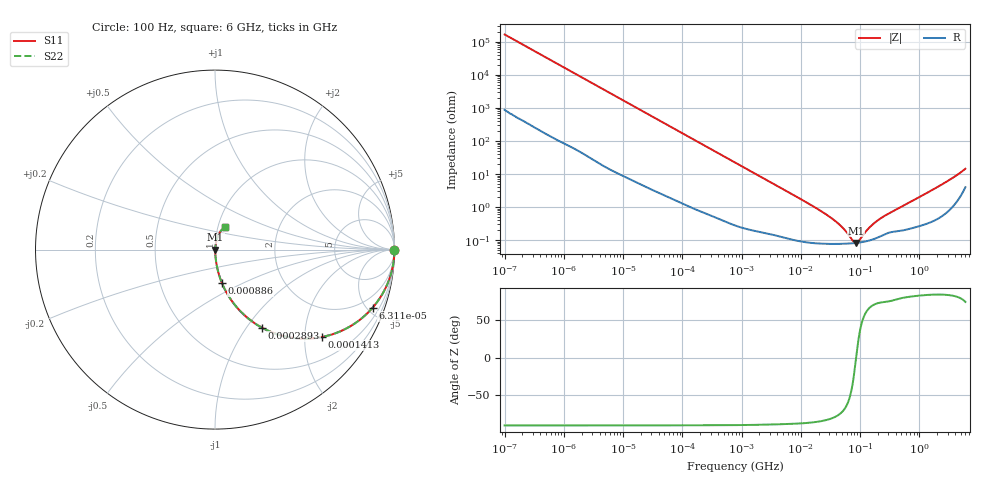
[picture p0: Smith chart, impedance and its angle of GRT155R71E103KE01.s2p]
!Murata Part Number: GRT155R71E103KE01
!These Parameters are Measured in Series Mode Connection
!Data Generated on Jun 19, 2026
!  o--ll--o
!Port1  Port2
!  o------o
!Operation Temp=25[degC], DC Bias Voltage=0[V]
!Freq. Start=100[Hz] Stop=6[GHz] 401[Steps]
# Hz S RI R 50
!Freq.(Hz) S11(Real) S11(Imag) S21(Real) S21(Imag) S12(Real) S12(Imag) S22(Real) S22(Imag)
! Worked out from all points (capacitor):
!   401 points, 100 Hz to 6 GHz, reference 50 ohm
!   read as one part in series: C = 9.51 nF near 109 Hz
!   lowest |Z| = 82.6 mohm at 85.28 MHz (marker M1)
!   series resonance near 85.79 MHz, so ESL is about 360 pH
!   S11 on the Smith chart (normalised r, x): 100 Hz: open; 63.12 kHz: 1.04, -5.41; 141.3 kHz: 1.02, -2.42; 289.3 kHz: 1.01, -1.19; 886 kHz: 1.01, -0.39; 6 GHz: 1.08, +0.28
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100  1 -0.000598  3.5e-06 0.000598  3.5e-06 0.000598  1 -0.000598
2008  0.9998 -0.0119  0.000204 0.0119  0.000204 0.0119  0.9998 -0.0119
12041  0.9946 -0.0706  0.00539 0.0706  0.00539 0.0706  0.9946 -0.0706
40335  0.9456 -0.2236  0.0544 0.2236  0.0544 0.2236  0.9456 -0.2236
63115  0.8779 -0.3239  0.1221 0.3239  0.1221 0.3239  0.8779 -0.3239
141303  0.5942 -0.4871  0.4058 0.4871  0.4058 0.4871  0.5942 -0.4871
289253  0.2629 -0.4354  0.7371 0.4354  0.7371 0.4354  0.2629 -0.4354
452617  0.1292 -0.3301  0.8708 0.3301  0.8708 0.3301  0.1292 -0.3301
774597  0.0498 -0.2113  0.9502 0.2113  0.9502 0.2113  0.0498 -0.2113
885955  0.039 -0.187  0.961 0.187  0.961 0.187  0.039 -0.187
2713602  0.00567 -0.0637  0.9943 0.0637  0.9943 0.0637  0.00567 -0.0637
1.555665e7  0.000943 -0.011  0.9991 0.011  0.9991 0.011  0.000943 -0.011
3.983537e7  0.000783 -0.00349  0.9992 0.00349  0.9992 0.00349  0.000783 -0.00349
5.449875e7  0.000784 -0.00194  0.9992 0.00194  0.9992 0.00194  0.000784 -0.00194
7.455971e7  0.000807 -0.00058  0.9992 0.00058  0.9992 0.00058  0.000807 -0.00058
8.527865e7  0.000825 -2.43e-05  0.9992 2.43e-05  0.9992 2.43e-05  0.000825 -2.43e-05
9.753859e7  0.00085 0.000529  0.9991 -0.000529  0.9991 -0.000529  0.00085 0.000529
1.275994e8  0.00093 0.00167  0.9991 -0.00167  0.9991 -0.00167  0.00093 0.00167
1.669249e8  0.00107 0.0029  0.9989 -0.0029  0.9989 -0.0029  0.00107 0.0029
3.124326e8  0.00174 0.00629  0.9983 -0.00629  0.9983 -0.00629  0.00174 0.00629
1.95892e9  0.00571 0.0386  0.9943 -0.0386  0.9943 -0.0386  0.00571 0.0386
6e9  0.0556 0.127  0.9444 -0.127  0.9444 -0.127  0.0556 0.127
